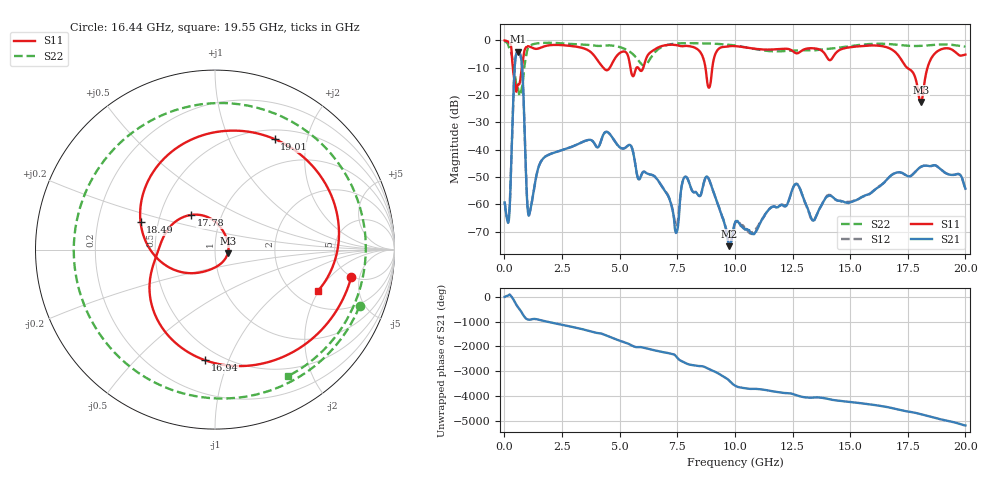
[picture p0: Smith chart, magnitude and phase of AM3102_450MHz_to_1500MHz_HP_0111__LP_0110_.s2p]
!Agilent Technologies,E8364B,MY43040894,A.07.50.67
!Agilent E8364B: A.07.50.67
!Date: Thursday, January 11, 2018 05:52:27
!Correction: S11(Full 2 Port(1,2))
!S21(Full 2 Port(1,2))
!S12(Full 2 Port(1,2))
!S22(Full 2 Port(1,2))
!S2P File: Measurements: S11, S21, S12, S22:
# Hz S  dB  R 50
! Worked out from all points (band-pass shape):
!   1601 points, 10 MHz to 20 GHz, reference 50 ohm
!   highest |S21| = -4.12 dB at 584.7 MHz (marker M1); lowest = -75.2 dB at 9.755 GHz (marker M2)
!   |S21| within 3 dB of the highest: 473.2 MHz to 735.4 MHz (262.2 MHz wide, 43.4 % of centre)
!   lowest |S11| = -22.6 dB at 18.06 GHz (marker M3), VSWR 1.16, Z = 57.6 - j2.47 ohm
!   |S11| at or under -10 dB: 365.4 MHz to 757.4 MHz (392 MHz wide, 69.8 % of centre); 8.723 GHz to 9.02 GHz (297 MHz wide, 3.35 % of centre); 17.47 GHz to 18.36 GHz (887.7 MHz wide, 4.96 % of centre)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
!   |S22| runs from -20.3 to -0.4 dB; largest |S21 - S12| = 0.0012
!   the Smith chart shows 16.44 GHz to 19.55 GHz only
!   S11 on the Smith chart (normalised r, x): 16.44 GHz: 4.90, -3.77; 16.94 GHz: 0.41, -0.83; 17.78 GHz: 0.71, +0.29; 18.49 GHz: 0.40, +0.15; 19.01 GHz: 0.62, +1.49; 19.55 GHz: 2.62, -1.95
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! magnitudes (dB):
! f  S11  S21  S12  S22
! 10 MHz  -0.1  -59.3  -59.2  -0.4
! 197.4 MHz  -0.7  -65.5  -64.7  -2.6
! 584.7 MHz  -16.2  -4.1  -4.1  -17.5
! 1.084 GHz  -2.3  -63.7  -63.2  -2.2
! 3.346 GHz  -2.7  -37.3  -37.3  -1.5
! 6.682 GHz  -2.6  -51.4  -51.4  -3.2
! 7.469 GHz  -1.8  -70.3  -68.1  -1.2
! 7.806 GHz  -2.1  -50.1  -50.3  -1.1
! 8.818 GHz  -16.2  -50.0  -50.0  -1.2
! 9.755 GHz  -2.2  -75.2  -74.6  -1.6
! 10.01 GHz  -2.1  -66.7  -67.0  -1.9
! 12.67 GHz  -4.7  -52.5  -52.4  -3.7
! 13.34 GHz  -2.9  -65.6  -65.6  -3.8
! 16.44 GHz  -2.2  -52.3  -52.3  -1.3
! 16.68 GHz  -2.8  -50.1  -50.2  -1.4
! 16.94 GHz  -4.2  -48.5  -48.6  -1.5
! 17.78 GHz  -12.6  -48.6  -48.5  -2.1
! 18.06 GHz  -22.6  -46.3  -46.3  -2.0
! 18.49 GHz  -7.1  -46.0  -46.0  -1.8
! 19.01 GHz  -3.1  -47.7  -47.8  -1.5
! 19.55 GHz  -4.2  -49.1  -49.1  -1.8
! 20 GHz  -5.2  -54.2  -54.3  -2.3
